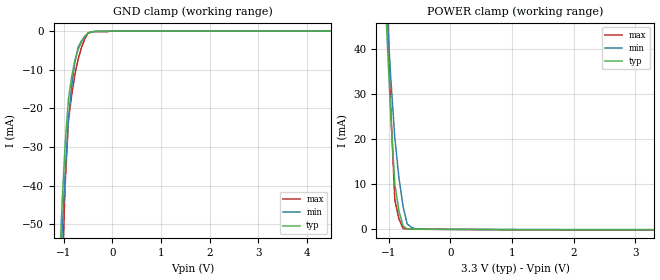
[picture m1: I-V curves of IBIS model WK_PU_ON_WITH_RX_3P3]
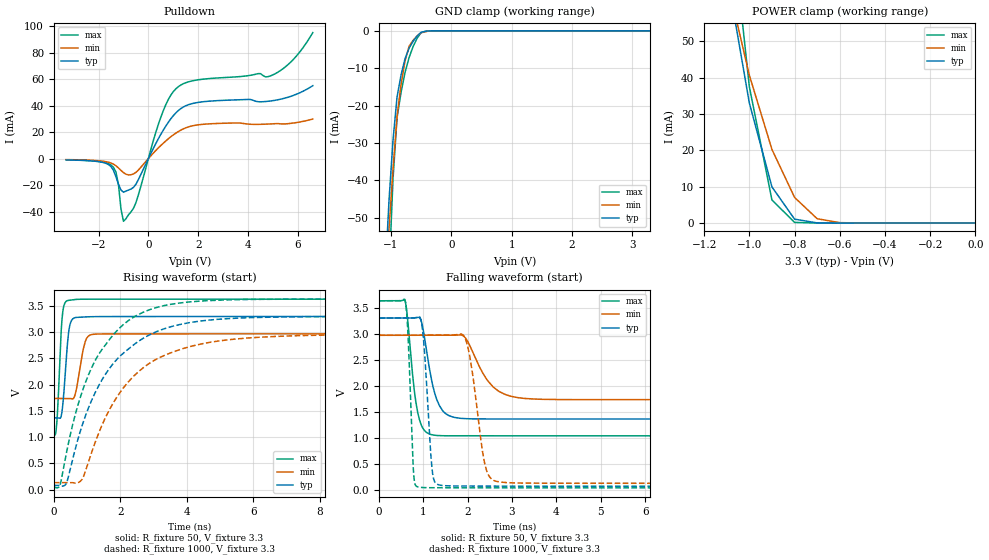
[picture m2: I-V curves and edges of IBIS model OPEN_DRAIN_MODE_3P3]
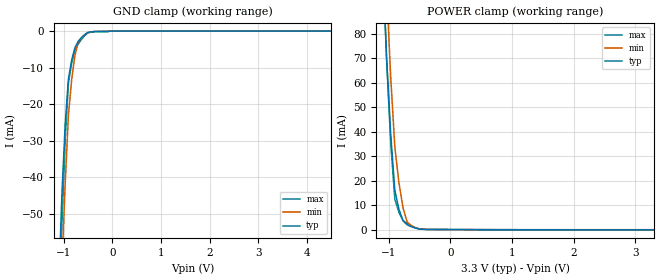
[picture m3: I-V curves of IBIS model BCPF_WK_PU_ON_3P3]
[IBIS Ver]   4.1
[File Name]   sprm822.ibs
[File Rev]   1.0
[Date]   AUG 26, 2022
[Source]   File originated at Texas Instruments
[Copyright]   (c) 2012, Texas Instruments Inc.
[Component]   f280013xrgz
[Manufacturer] Texas Instruments
[Package]
| Variable   Typ   Min   Max
R_pkg   0.2239	0.1212   0.2900
L_pkg   3.1309E-09	2.4320E-09	3.7950E-09
C_pkg   0.1501E-12	0.1260E-12	0.1886E-12
[Pin]   signal_name   model_name   R_pin   L_pin   C_pin
1	GPIO29	BCF3385DSHYPBFZ_LC_IOTB_USF	0.254	3.5105E-09	0.1288E-12
2	GPIO28	BCF3385DSHYPBFZ_LC_IOTB_USF	0.2317	3.1951E-09	0.1522E-12
3	XRSn	BQ0491FS_CORNER_USF	0.2221	3.0288E-09	0.148E-12
4	GPIO228/GPIO226	BCF3385DSHYPBFZ_LC_IOTB_USF	0.2181	3.0477E-09	0.1609E-12
5	GPIO242	BCF3385DSHYPBFZ_LC_IOTB_USF	0.2196	2.9223E-09	0.1475E-12
6	GPIO224	BCF3385DSHYPBFZ_LC_IOTB_USF	0.2131	2.8476E-09	0.1434E-12
7	A15/C7/CMP1/C4/A14/ADCINCAL/CMP3P	ICF33SHYPB_LC_IOTB	0.2015	2.833E-09	0.153E-12
8	A11/C0/CMP1/TESTANA0	ICF33SHYPB_LC_IOTB	0.213	2.8536E-09	0.1471E-12
9	A5/C2/CMP3	ICF33SHYPB_LC_IOTB	2.20E-01	2.9406E-09	0.1491E-12
10	A1/CMP1P	ICF33SHYPB_LC_IOTB	2.33E-01	3.108E-09	0.1529E-12
11	A0/C15/CMP3P/DACOUT	ICF33SHYPB_LC_IOTB	2.54E-01	3.338E-09	0.1582E-12
12	VREFHIAC	NC	1.50E-01	3.0841E-09	0.1483E-12
13	VREFLOAC	NC	1.50E-01	3.1775E-09	0.1423E-12
14	A12/C1/TESTANA1/CMP2/CMP4P	ICF33SHYPB_LC_IOTB	2.46E-01	3.3326E-09	0.1527E-12
15	A7/C3/CMP4	ICF33SHYPB_LC_IOTB	2.18E-01	2.9893E-09	0.1479E-12
16	A8/C11/CMP2P/CMP4P	ICF33SHYPB_LC_IOTB	2.18E-01	2.907E-09	0.1479E-12
17	VSSA	NC	1.25E-01	2.4986E-09	0.1583E-12
18	VDDA	NC	1.27E-01	2.5288E-09	0.159E-12
19	A4/C14/CMP2P/CMP4	ICF33SHYPB_LC_IOTB	2.43E-01	3.0765E-09	0.1497E-12
20	GPIO227	BCF3385DSHYPBFZ_LC_IOTB_USF	2.45E-01	3.1431E-09	0.1499E-12
21	GPIO230	BCF3385DSHYPBFZ_LC_IOTB_USF	2.64E-01	3.3646E-09	0.1544E-12
22	GPIO13	BCF3385DSHYPBFZ_LC_IOTB_USF	2.65E-01	3.4422E-09	0.156E-12
23	GPIO12	BCF3385DSHYPBFZ_LC_IOTB_USF	2.90E-01	3.7399E-09	0.1614E-12
24	GPIO33	BCF3385DSHYPBFZ_LC_IOTB_USF	2.55E-01	3.5479E-09	0.1272E-12
25	GPIO16	BCF3385DSHYPBFZ_LC_IOTB_USF	2.48E-01	3.4987E-09	0.1266E-12
26	GPIO24	BCF3385DSHYPBFZ_LC_IOTB_USF	2.33E-01	3.2396E-09	0.1497E-12
27	JTAG_TCK	BCF3355DSHYPBFZ_TMS_USF	2.17E-01	3.0096E-09	0.1467E-12
28	GPIO37/TDO	BCPF335585DSHYPBFZ_LC_IOTB_USF	2.12E-01	2.9113E-09	0.1446E-12
29	JTAG_TMS	BCF3355DSHYPBFZ_TMS_USF	2.12E-01	2.8701E-09	0.1448E-12
30	GPIO35/TDI	BCF3385DSHYPBFZ_LC_IOTB_USF	2.19E-01	2.908E-09	0.1457E-12
31	GPIO32	BCF3385DSHYPBFZ_LC_IOTB_USF	2.29E-01	3.0073E-09	0.1484E-12
32	GPIO18/X2	BCF3385DSHYPBFZ_LC_IOTB_USF	2.36E-01	3.1782E-09	0.1653E-12
33	GPIO19/X1/ExtR	BCPF335585DSHYPBFZ_LC_IOTB_USF	2.66E-01	3.4708E-09	0.1802E-12
34	VDDSFL	NC	2.75E-01	3.5793E-09	0.188E-12
35	VDD	NC	1.53E-01	3.1025E-09	0.1887E-12
36	GPIO8	BCF3385DSHYPBFZ_LC_IOTB_USF	2.48E-01	3.4969E-09	0.1274E-12
37	GPIO4	BCF3385DSHYPBFZ_LC_IOTB_USF	2.81E-01	3.795E-09	0.1345E-12
38	GPIO3	BCF3385DSHYPBFZ_LC_IOTB_USF	2.64E-01	3.5251E-09	0.1555E-12
39	GPIO2	BCF3385DSHYPBFZ_LC_IOTB_USF	2.49E-01	3.3047E-09	0.153E-12
40	GPIO1	BCF3385DSHYPBFZ_LC_IOTB_USF	2.32E-01	3.0889E-09	0.1501E-12
41	GPIO0	BCF3385DSHYPBFZ_LC_IOTB_USF	2.20E-01	2.9395E-09	0.1457E-12
42	GPIO23	BCF3385DSHYPBFZ_LC_IOTB_USF	2.16E-01	2.8812E-09	0.142E-12
43	GPIO7	BCF3385DSHYPBFZ_LC_IOTB_USF	2.16E-01	2.86E-09	0.1433E-12
44	VDD	NC	1.21E-01	2.432E-09	0.1574E-12
45	VDDSFL	NC	2.23E-01	2.9776E-09	0.1472E-12
46	GPIO5	BCF3385DSHYPBFZ_LC_IOTB_USF	2.24E-01	3.0545E-09	0.1499E-12
47	GPIO9	BCF3385DSHYPBFZ_LC_IOTB_USF	2.38E-01	3.2597E-09	0.1517E-12
48	GPIO6	BCF3385DSHYPBFZ_LC_IOTB_USF	2.45E-01	3.4369E-09	0.126E-12
| End of package information
|   Component BQ0491FS_CORNER_USF
[Component]   BQ0491FS_CORNER_USF
[Manufacturer]   Texas Instruments
[Package]
|  variable   typ   min   max
R_pkg   0   0   0
L_pkg   0   0   0
C_pkg   0   0   0
[Pin]   signal_name   model_name   R_pin   L_pin   C_pin
VSS   VSS   GND
VDDS   VDDS   POWER
PAD   PAD   BQ0491FS_CORNER_USF
[Model Selector] BQ0491FS_CORNER_USF
WK_PU_ON_WITH_RX_3P3  Cell operated at 3.3(nom)
|WK_PU_ON_WITH_RX_3P3; WEAK_PULLUP_ON_WITH_RX
OPEN_DRAIN_MODE_3P3  Cell operated at 3.3(nom)
|   Component BCPF335585DSHYPBFZ_LC_IOTB_USF
[Component]   BCPF335585DSHYPBFZ_LC_IOTB_USF
[Manufacturer]   Texas Instruments
[Package]
|  variable   typ   min   max
R_pkg   0   0   0
L_pkg   0   0   0
C_pkg   0   0   0
[Pin]   signal_name   model_name   R_pin   L_pin   C_pin
VSS   VSS   GND
VDDS   VDDS   POWER
PAD   PAD   BCPF335585DSHYPBFZ_LC_IOTB_USF
[Model Selector] BCPF335585DSHYPBFZ_LC_IOTB_USF
BCPF_WK_PU_ON_3P3  Cell operated at 3.3(nom)
|BCPF_WK_PU_ON_3P3; WEAK_PULLUP_ON
BCPF_DRIVER_MODE_4MA_3P3  Cell operated at 3.3(nom)
|BCPF_DRIVER_MODE_4MA_3P3
BCPF_DRIVER_MODE_2MA_3P3  Cell operated at 3.3(nom)
|BCPF_DRIVER_MODE_2MA_3P3
BCPF_WK_PD_ON_3P3  Cell operated at 3.3(nom)
|   Component ICF33SHYPB_LC_IOTB
[Component]   ICF33SHYPB_LC_IOTB
[Manufacturer]   Texas Instruments
[Package]
|  variable   typ   min   max
R_pkg   0   0   0
L_pkg   0   0   0
C_pkg   0   0   0
[Pin]   signal_name   model_name   R_pin   L_pin   C_pin
VSS   VSS   GND
VDDS   VDDS   POWER
PAD   PAD   ICF33SHYPB_LC_IOTB
[Model Selector] ICF33SHYPB_LC_IOTB
ICF_RECEIVER_MODE_3P3  Cell operated at 3.3(nom)
|ICF_RECEIVER_MODE_3P3; RECEIVER_MODE
ICF_WK_PU_ON_3P3  Cell operated at 3.3(nom)
|ICF_WK_PU_ON_3P3; WEAK_PULLUP_ON
ICF_WK_PD_ON_3P3  Cell operated at 3.3(nom)
|   Component BCF3385DSHYPBFZ_LC_IOTB_USF
[Component]   BCF3385DSHYPBFZ_LC_IOTB_USF
[Manufacturer]   Texas Instruments
[Package]
|  variable   typ   min   max
R_pkg   0   0   0
L_pkg   0   0   0
C_pkg   0   0   0
[Pin]   signal_name   model_name   R_pin   L_pin   C_pin
VSS   VSS   GND
VDDS   VDDS   POWER
PAD   PAD   BCF3385DSHYPBFZ_LC_IOTB_USF
[Model Selector] BCF3385DSHYPBFZ_LC_IOTB_USF
BCF_WK_PU_ON_3P3  Cell operated at 3.3(nom)
|BCF_WK_PU_ON_3P3; WEAK_PULLUP_ON
BCF_WK_PD_ON_3P3  Cell operated at 3.3(nom)
|BCF_WK_PD_ON_3P3; WEAK_PULLDOWN_ON
BCF_DRIVER_MODE_3P3  Cell operated at 3.3(nom)
|BCF_DRIVER_MODE_3P3
BCF_RECEIVER_MODE_3P3  Cell operated at 3.3(nom)
|   Component BCF3355DSHYPBFZ_TMS_USF
[Component]   BCF3355DSHYPBFZ_TMS_USF
[Manufacturer]   Texas Instruments
[Package]
|  variable   typ   min   max
R_pkg   0   0   0
L_pkg   0   0   0
C_pkg   0   0   0
[Pin]   signal_name   model_name   R_pin   L_pin   C_pin
VSS   VSS   GND
VDDS   VDDS   POWER
PAD   PAD   BCF3355DSHYPBFZ_TMS_USF
[Model Selector] BCF3355DSHYPBFZ_TMS_USF
TMS_WK_PU_ON_3P3  Cell operated at 3.3(nom)
|TMS_WK_PU_ON_3P3; WEAK_PULLUP_ON
TMS_DRIVER_3P3  Cell operated at 3.3(nom)
|TMS_DRIVER_3P3
TMS_WK_PD_ON_3P3  Cell operated at 3.3(nom)
| Models and submodels in the file (16): WK_PU_ON_WITH_RX_3P3 (Input), OPEN_DRAIN_MODE_3P3 (I/O_open_drain), BCPF_WK_PU_ON_3P3 (Input), BCPF_DRIVER_MODE_4MA_3P3 (I/O), BCPF_DRIVER_MODE_2MA_3P3 (I/O), BCPF_WK_PD_ON_3P3 (Input), ICF_RECEIVER_MODE_3P3 (Input), ICF_WK_PU_ON_3P3 (Input), ICF_WK_PD_ON_3P3 (Input), BCF_WK_PU_ON_3P3 (Input), BCF_WK_PD_ON_3P3 (Input), BCF_DRIVER_MODE_3P3 (I/O), BCF_RECEIVER_MODE_3P3 (Input), TMS_WK_PU_ON_3P3 (Input), TMS_DRIVER_3P3 (I/O), TMS_WK_PD_ON_3P3 (Input)
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|OPEN_DRAIN_MODE_3P3
|   Model Cell WK_PU_ON_WITH_RX_3P3
|WK_PU_ON_WITH_RX_3P3
[Model]   WK_PU_ON_WITH_RX_3P3
Model_type   Input
Polarity   Non-Inverting
Vinl =  0.8
Vinh =  2
C_comp   1.11773p   1.013376p   1.244487p
[Model Spec]
Vinl   0.8   0.8   0.8
Vinh   2   2   2
[Temperature Range]   25   155   -40
[Voltage Range]   3.3   2.97   3.63
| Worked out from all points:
|   GND clamp passes 1 mA (typ) near -0.54 V on its own axis
|   POWER clamp passes 1 mA (typ) near -0.77 V on its own axis
| Nom Voltages:
|   BIASFET=3.3, VDD=1.2, VDDS=3.3, VSS=0
| Min Voltages:
|   BIASFET=2.97, VDD=1.08, VDDS=2.97, VSS=0
| Max Voltages:
|   BIASFET=3.63, VDD=1.32, VDDS=3.63, VSS=0
[POWER_clamp]
|   voltage   I(typ)   I(min)   I(max)
-3.3V     1.132A     1.059A     1.769A
-1.033V   45.08mA    49.59mA    56.93mA
-966.7mV  25.39mA    33.9mA     27.23mA
-900mV    10.01mA    20.29mA    6.454mA
-833.3mV  4.092mA    11.48mA    2.326mA
-766.7mV  785.4uA    5.125mA    201.1uA
-700mV    89.29uA    1.212mA    78.7uA
-633.3mV  61.2uA     494uA      69.62uA
-566.7mV  44.07uA    99.73uA    61.24uA
3.3V      -85.93uA   -55.95uA   -137.9uA
[GND_clamp]
|   voltage   I(typ)   I(min)   I(max)
-3.3V     -1.198A    -966mA     -2.548A
-1.1V     -66.27mA   -70.87mA   -99.83mA
-1.033V   -45.41mA   -52.93mA   -65.12mA
-966.7mV  -29.23mA   -36.93mA   -39.6mA
-900mV    -17.72mA   -22.86mA   -23.27mA
-833.3mV  -11.83mA   -14.27mA   -16.55mA
-766.7mV  -7.493mA   -8.038mA   -11.21mA
-700mV    -4.704mA   -4.168mA   -7.263mA
-566.7mV  -1.465mA   -1.376mA   -2.095mA
-500mV    -469.8uA   -575.8uA   -591.3uA
-33.33mV  0A         0A         0A
6.6V      0A         0A         0A
|   Model Cell OPEN_DRAIN_MODE_3P3
|OPEN_DRAIN_MODE_3P3
[Model]   OPEN_DRAIN_MODE_3P3
Model_type   I/O_open_drain
Polarity   Non-Inverting
Enable   Active-Low
Vinl =  0.8
Vinh =  2
Cref =  15.0000pF
Rref =  100.0000M
Vref =  0V
Vmeas =  1.65
C_comp   1.11773p   1.013376p   1.244487p
[Model Spec]
Vinl   0.8   0.8   0.8
Vinh   2   2   2
[Temperature Range]   25   155   -40
[Voltage Range]   3.3   2.97   3.63
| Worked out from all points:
|   slope of the pulldown table from 0 to 0.495 V, typ, clamps not added: 27.3 ohm
|   GND clamp passes 1 mA (typ) near -0.54 V on its own axis
|   POWER clamp passes 1 mA (typ) near -0.79 V on its own axis
|   rising waveform, R_fixture 50, V_fixture 3.3: 20-80 % time 139ps typ, 204ps min, 112ps max; typ from 1.37 V to 3.3 V
|   rising waveform, R_fixture 1000, V_fixture 3.3: 20-80 % time 1.57ns typ, 1.73ns min, 1.34ns max; typ from 0.081 V to 3.3 V
|   falling waveform, R_fixture 50, V_fixture 3.3: 20-80 % time 266ps typ, 495ps min, 195ps max; typ from 3.3 V to 1.37 V
|   falling waveform, R_fixture 1000, V_fixture 3.3: 20-80 % time 138ps typ, 264ps min, 97ps max; typ from 3.3 V to 0.081 V
| Nom Voltages:
|   BIASFET=3.3, VDD=1.2, VDDS=3.3, VSS=0
| Min Voltages:
|   BIASFET=2.97, VDD=1.08, VDDS=2.97, VSS=0
| Max Voltages:
|   BIASFET=3.63, VDD=1.32, VDDS=3.63, VSS=0
[POWER_clamp]
|   voltage   I(typ)   I(min)   I(max)
-3.3V     1.132A     1.059A     1.769A
-1.067V   57.04mA    58.46mA    76.19mA
-1.033V   45.04mA    49.58mA    56.86mA
-1V       33.04mA    40.7mA     37.54mA
-900mV    9.95mA     20.27mA    6.36mA
-800mV    1.073mA    7.058mA    176.5uA
-700mV    35.88uA    1.186mA    3.424uA
-600mV    1.374uA    110.7uA    455.3nA
0V        338.2pA    5.96nA     285.2pA
[Pulldown]
|   voltage   I(typ)   I(min)   I(max)
-3.3V     -1.018mA   -784.1uA   -895.6uA
-1.4V     -8.945mA   -4.198mA   -6.606mA
-1.2V     -19.44mA   -7.097mA   -19.74mA
-1.1V     -23.79mA   -8.926mA   -38.1mA
-1V       -25.42mA   -10.61mA   -47.4mA
-500mV    -19.36mA   -10.45mA   -33.38mA
500mV     18.33mA    9.885mA    31.3mA
1.1V      34.47mA    19.21mA    52.67mA
2.1V      42.73mA    25.73mA    59.79mA
4.9V      43.52mA    26.17mA    62.49mA
5.8V      47.6mA     26.81mA    74.57mA
6.6V      55.08mA    29.87mA    95.23mA
[GND_clamp]
|   voltage   I(typ)   I(min)   I(max)
-3.3V     -1.198A    -966mA     -2.548A
-1.1V     -66.26mA   -70.86mA   -99.82mA
-1.033V   -45.39mA   -52.93mA   -65.1mA
-966.7mV  -29.21mA   -36.92mA   -39.58mA
-900mV    -17.69mA   -22.85mA   -23.24mA
-833.3mV  -11.79mA   -14.25mA   -16.46mA
-766.7mV  -7.428mA   -8.019mA   -11.09mA
-700mV    -4.622mA   -4.142mA   -7.129mA
-566.7mV  -1.379mA   -1.338mA   -1.958mA
-500mV    -383.7uA   -535.9uA   -452.8uA
-300mV    -821.5nA   -7.147uA   -404.1nA
3.3V      338.2pA    143.1nA    239.5pA
[Ramp]
| variable   typ   min   max
dV/dt_f  1.1674782/0.26758435n 0.74431688/0.49748067n  1.5612158/0.19548637n
dV/dt_r 16.566269m/0.16851048n 10.821448m/0.18717204n 21.089911m/0.14213015n
R_load = 50
[Rising Waveform]
R_fixture = 50
V_fixture = 3.3
V_fixture_min = 2.97
V_fixture_max = 3.63
|   time   V(typ)   V(min)   V(max)
0s        1.368V     1.738V     1.045V
85.1ps    1.368V     1.738V     1.237V
222.8ps   1.404V     1.738V     3.038V
302.4ps   1.849V     1.738V     3.503V
480.8ps   3.134V     1.739V     3.611V
650.9ps   3.28V      1.835V     3.625V
883.3ps   3.29V      2.667V     3.629V
1.085ns   3.296V     2.946V     3.63V
2.138ns   3.3V       2.969V     3.63V
500ns     3.3V       2.97V      3.63V
[Rising Waveform]
R_fixture = 1000
V_fixture = 3.3
V_fixture_min = 2.97
V_fixture_max = 3.63
|   time   V(typ)   V(min)   V(max)
0s        81.2mV     135.1mV    50.52mV
192.5ps   77.67mV    135.1mV    97.37mV
387.1ps   134.1mV    135mV      724.8mV
838.5ps   1.197V     186.7mV    1.84V
1.379ns   2.014V     1.122V     2.607V
1.98ns    2.537V     1.841V     3.081V
2.544ns   2.825V     2.247V     3.337V
3.332ns   3.068V     2.56V      3.51V
5.837ns   3.277V     2.89V      3.625V
500ns     3.3V       2.97V      3.63V
[Falling Waveform]
R_fixture = 50
V_fixture = 3.3
V_fixture_min = 2.97
V_fixture_max = 3.63
|   time   V(typ)   V(min)   V(max)
0s        3.3V       2.97V      3.63V
583ps     3.3V       2.97V      3.638V
803.8ps   3.302V     2.97V      1.863V
915.1ps   3.309V     2.97V      1.349V
1.254ns   1.867V     2.97V      1.057V
1.503ns   1.472V     2.97V      1.047V
1.948ns   1.375V     2.922V     1.047V
2.701ns   1.368V     1.897V     1.046V
4.266ns   1.368V     1.739V     1.045V
500ns     1.368V     1.738V     1.045V
[Falling Waveform]
R_fixture = 1000
V_fixture = 3.3
V_fixture_min = 2.97
V_fixture_max = 3.63
|   time   V(typ)   V(min)   V(max)
0s        3.3V       2.97V      3.63V
597.9ps   3.3V       2.97V      3.609V
783.5ps   3.301V     2.97V      294.5mV
944.1ps   3.272V     2.97V      59.09mV
1.149ns   937.5mV    2.97V      52.6mV
1.266ns   149.7mV    2.97V      52.01mV
1.948ns   84.58mV    2.907V     50.29mV
2.499ns   83.13mV    253.5mV    50.07mV
3.393ns   81.49mV    140.3mV    50.06mV
500ns     81.2mV     135.1mV    50.06mV
|BCPF_WK_PD_ON_3P3; WEAK_PULLDOWN_ON
|   Model Cell BCPF_WK_PU_ON_3P3
|BCPF_WK_PU_ON_3P3
[Model]   BCPF_WK_PU_ON_3P3
Model_type   Input
Polarity   Non-Inverting
Vinl =  0.8
Vinh =  2
C_comp   1.21982p   0.982413p   1.3757p
[Model Spec]
Vinl   0.8   0.8   0.8
Vinh   2   2   2
[Temperature Range]   25   155   -40
[Voltage Range]   3.3   2.97   3.63
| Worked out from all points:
|   GND clamp passes 1 mA (typ) near -0.57 V on its own axis
|   POWER clamp passes 1 mA (typ) near -0.61 V on its own axis
| Nom Voltages:
|   BIASFET=3.3, VDD=1.2, VDDS=3.3, VSS=0
| Min Voltages:
|   BIASFET=2.97, VDD=1.08, VDDS=2.97, VSS=0
| Max Voltages:
|   BIASFET=3.63, VDD=1.32, VDDS=3.63, VSS=0
[POWER_clamp]
|   voltage   I(typ)   I(min)   I(max)
-3.3V     1.919A     2.431A     2.069A
-1.1V     109.8mA    140.8mA    113.2mA
-1.033V   70.21mA    98.04mA    69.24mA
-966.7mV  38.95mA    62.35mA    35.63mA
-900mV    16.03mA    33.73mA    12.36mA
-833.3mV  8.266mA    19.09mA    7.029mA
-766.7mV  3.571mA    8.879mA    3.722mA
-700mV    1.939mA    3.079mA    2.444mA
-566.7mV  603.9uA    711.2uA    759.2uA
-500mV    195.8uA    269.7uA    227.2uA
-366.7mV  40.85uA    44.56uA    53.2uA
3.3V      -108.8uA   -62.99uA   -174uA
[GND_clamp]
|   voltage   I(typ)   I(min)   I(max)
-3.3V     -1.48A     -1.41A     -2.182A
-1.1V     -69.91mA   -89.89mA   -82.68mA
-1.033V   -44.46mA   -64.18mA   -52.64mA
-966.7mV  -25.52mA   -41.89mA   -29.83mA
-900mV    -13.08mA   -23mA      -14.24mA
-833.3mV  -7.945mA   -13.29mA   -8.83mA
-766.7mV  -4.523mA   -6.66mA    -5.269mA
-700mV    -2.817mA   -3.105mA   -3.556mA
-566.7mV  -980.5uA   -1.002mA   -1.249mA
-500mV    -376.2uA   -438.1uA   -476.5uA
-33.33mV  0A         0A         0A
6.6V      0A         0A         0A
